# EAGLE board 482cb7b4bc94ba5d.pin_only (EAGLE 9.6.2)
REV: D

Size 25.4 x 17.78 mm. Coordinates in mm from the lower left corner, seen from the top.
Outline: 0,15.24 0,2.54 arc90 2.54,0 22.86,0 arc90 25.4,2.54 25.4,15.24 arc90 22.86,17.78 2.54,17.78 arc90 0,15.24
Copper layers (1*16): Top 0.035mm / dielectric 1.5mm / Bottom 0.035mm
Design rules "adafruit *": minimum track width 8mil, minimum drill 15.5mil, track to track 8mil, track to pad 8mil, pad to pad 8mil, via to via 8mil, smd to smd 8mil, copper to edge 10mil, drill to drill 8mil, minimum pad ring 10mil, minimum via ring 8mil, stop-mask expansion 2mil, vias tented up to drill 20mil, thermal gap 10mil
Net classes: 1 highpower: width 0.305 mm, drill 0.483 mm; 2 lowpower: width 0.305 mm, drill 0.483 mm
Holes 2.54 mm at 2.54,2.54 22.86,2.54

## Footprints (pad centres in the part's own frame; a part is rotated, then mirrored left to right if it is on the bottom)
0603-NO = smd 1.075 x 1: 1 -0.85,0; 2 0.85,0
0805-NO = smd 1.24 x 1.5: 1 -0.95,0; 2 0.95,0
JST_SH4 = smd 0.6 x 1.55: 1 -1.5,2.514; 2 -0.5,2.514; 3 0.5,2.514; 4 1.5,2.514 | smd 1.2 x 1.8: MT1 -2.8,-1.386; MT2 2.8,-1.386
CHIPLED_0603_NOOUTLINE = smd 0.8 x 0.8: A 0,-0.75; C 0,0.75
SOD-323 = smd 1.35 x 0.8: A 1.27,0; C -1.27,0
FIDUCIAL_1MM = smd 1 x 1: 1 0,0
BME680 = smd 0.4 x 0.4: 1 1.2,1.2; 2 1.2,0.4; 3 1.2,-0.4; 4 1.2,-1.2; 5 -1.2,-1.2; 6 -1.2,-0.4; 7 -1.2,0.4; 8 -1.2,1.2
1X07_ROUND_70 = drill 1 pad 1.778: 1 -7.62,0; 2 -5.08,0; 3 -2.54,0; 4 0,0; 5 2.54,0; 6 5.08,0; 7 7.62,0
SOT363 = smd 0.5 x 0.5: 1 -0.75,-0.9; 3 0.75,-0.9; 4 0.75,0.9; 6 -0.75,0.9 | smd 0.4 x 0.5: 2 0,-0.9; 5 0,0.9
RESPACK_4X0603 = smd 0.45 x 0.9: 1 -1.3,-0.85; 2 -0.4,-0.85; 3 0.4,-0.85; 4 1.3,-0.85; 5 1.3,0.85; 6 0.4,0.85; 7 -0.4,0.85; 8 -1.3,0.85
SOLDERJUMPER_ARROW_NOPASTE = smd 0.762 x 1.524: 1 -1.016,0; 2 1.016,0
SOT23-5 = smd 0.55 x 1.2: 1 -0.95,-1.3; 2 0,-1.3; 3 0.95,-1.3; 4 0.95,1.3; 5 -0.95,1.3
MOUNTINGHOLE_2.5_PLATED = drill 2.5 pad 3.2: P$1 0,0

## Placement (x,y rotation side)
C1  0.1uF  [0603-NO]  10.03,8.92 270 top
C2  10uF  [0805-NO]  7.49,5.71 0 top
C3  10uF  [0805-NO]  8.13,12.19 0 top
CONN3  STEMMA_I2C_QT  [JST_SH4]  22.86,8.89 90 top
CONN4  STEMMA_I2C_QT  [JST_SH4]  2.54,8.89 270 top
D1  GREEN  [CHIPLED_0603_NOOUTLINE]  3.56,12.57 90 top
D2  1N4148  [SOD-323]  12.7,12.95 180 top
FID3  FIDUCIAL_1MM  [FIDUCIAL_1MM]  1.02,4.38 0 top
FID4  FIDUCIAL_1MM  [FIDUCIAL_1MM]  19.68,16.29 0 top
IC1  BME680  [BME680]  12.7,8.89 0 top
JP1  [1X07_ROUND_70]  12.7,2.54 0 top
Q2  BSS138  [SOT363]  17.02,7.49 90 top
R1  10K  [0603-NO]  5.59,12.45 270 top
R3  10K  [RESPACK_4X0603]  17.14,11.43 180 top
R4  10K  [0603-NO]  12.75,5.41 0 top
R5  10K  [0603-NO]  11.43,11.3 180 top
SJ1  [SOLDERJUMPER_ARROW_NOPASTE]  12.95,5.21 180 bottom
U2  AP2112K-3.3  [SOT23-5]  7.75,8.89 0 top
U$1  MOUNTINGHOLE2.5  [MOUNTINGHOLE_2.5_PLATED]  2.54,15.24 0 top
U$4  [ADAFRUIT_2.5MM]  4.7,15.11 0 top
U$17  MOUNTINGHOLE2.5  [MOUNTINGHOLE_2.5_PLATED]  22.86,15.24 0 top
U$25  [PCBFEAT-REV-040]  3.94,4.95 0 bottom
U$30  [STEMMAQT]  22.48,4.45 90 bottom
U$31  [STEMMAQT]  2.92,13.34 270 bottom

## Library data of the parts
C1-C3 CONN3 CONN4 D1 D2 JP1 Q2 R1 R3-R5 U2 U$4 U$25 = microbuilder
FID3 FID4 SJ1 U$1 U$17 = microbuilder; BOM: EXCLUDE
IC1 = adafruit_sensor
U$30 U$31 = silks

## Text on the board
tPlace: BME680 | Pres/Hum/Temp/Gas | on | 3Vo | SCK | SDI | VIN | GND | SDO | CS
bPlace: BME680 | Temp, Pressure / Humidity & Gas | Default I2C Addr 0x77 | Addr | VLogic/Vcc: 3-5VDC

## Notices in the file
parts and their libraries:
microbuilder: This work is placed in the public domain, and may be freely used for commercial and non-commercial work with the following conditions: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
